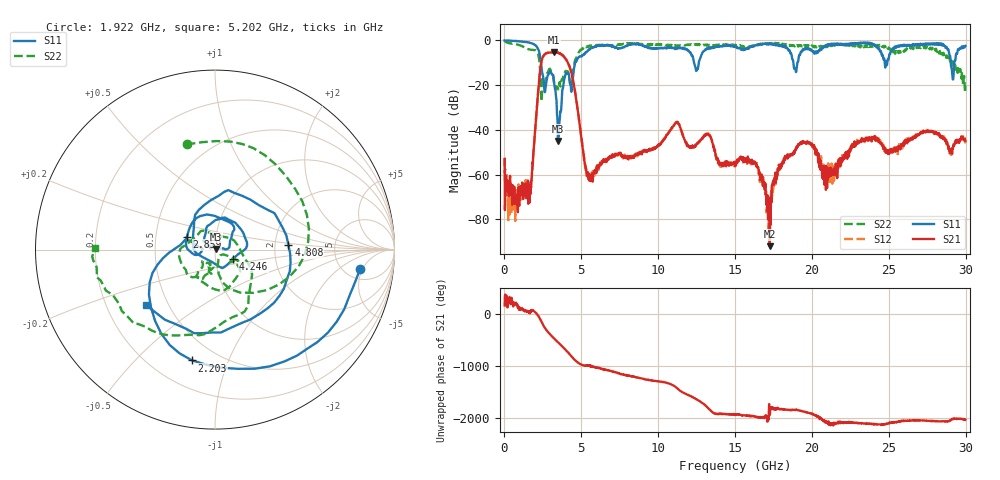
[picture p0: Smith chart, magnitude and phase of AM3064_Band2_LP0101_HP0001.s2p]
# Hz S DB R 50.0
!freq dBS11 angS11 dBS21 angS21 dBS12 angS12 dBS22 angS22
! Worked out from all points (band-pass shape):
!   1600 points, 10 MHz to 29.98 GHz, reference 50 ohm
!   highest |S21| = -5.14 dB at 3.215 GHz (marker M1); lowest = -92.1 dB at 17.25 GHz (marker M2)
!   |S21| within 3 dB of the highest: 2.46 GHz to 3.963 GHz (1.503 GHz wide, 46.8 % of centre)
!   lowest |S11| = -45.0 dB at 3.478 GHz (marker M3), VSWR 1.01, Z = 50.4 + j0.404 ohm
!   |S11| at or under -10 dB: 2.379 GHz to 4.595 GHz (2.216 GHz wide, 63.6 % of centre); 12.33 GHz to 12.64 GHz (312.3 MHz wide, 2.5 % of centre); 18.8 GHz to 19.05 GHz (253 MHz wide, 1.34 % of centre)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
!   |S22| runs from -27.3 to -0.2 dB; largest |S21 - S12| = 0.015
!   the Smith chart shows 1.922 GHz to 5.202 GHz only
!   S11 on the Smith chart (normalised r, x): 1.922 GHz: 6.83, -4.48; 2.203 GHz: 0.36, -0.75; 2.859 GHz: 0.72, +0.10; 4.246 GHz: 1.21, -0.13; 4.808 GHz: 2.38, +0.14; 5.202 GHz: 0.38, -0.31
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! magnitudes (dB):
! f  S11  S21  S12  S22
! 10 MHz  0.0  -53.1  -52.4  -0.2
! 572.3 MHz  -0.2  -72.9  -70.7  -1.5
! 1.547 GHz  -0.8  -73.1  -66.0  -3.9
! 1.922 GHz  -1.8  -46.7  -46.6  -4.3
! 2.203 GHz  -4.0  -22.2  -22.2  -6.5
! 2.859 GHz  -15.3  -5.5  -5.5  -13.7
! 3.215 GHz  -18.1  -5.1  -5.2  -18.2
! 3.478 GHz  -45.0  -5.5  -5.5  -21.4
! 4.246 GHz  -18.9  -11.8  -11.9  -17.9
! 4.808 GHz  -7.7  -33.3  -33.2  -5.6
! 5.015 GHz  -7.2  -44.1  -44.1  -4.2
! 5.202 GHz  -6.1  -53.6  -54.0  -3.5
! 10 GHz  -3.5  -46.7  -47.1  -1.9
! 11.24 GHz  -3.7  -36.7  -36.7  -2.6
! 15 GHz  -2.7  -56.4  -54.7  -2.0
! 16.35 GHz  -2.2  -54.9  -55.6  -2.4
! 17.25 GHz  -1.5  -92.1  -70.6  -1.3
! 18.25 GHz  -3.2  -51.7  -53.2  -1.8
! 19.99 GHz  -4.4  -46.7  -46.8  -2.3
! 20.97 GHz  -2.5  -58.5  -60.0  -2.5
! 25 GHz  -8.1  -49.3  -50.3  -3.2
! 29.98 GHz  -2.5  -44.8  -44.8  -20.2
